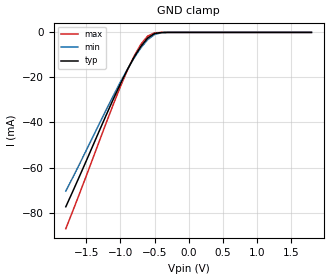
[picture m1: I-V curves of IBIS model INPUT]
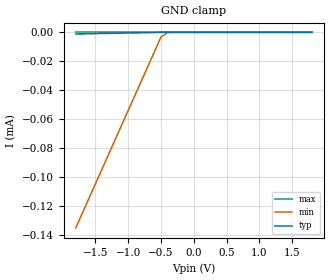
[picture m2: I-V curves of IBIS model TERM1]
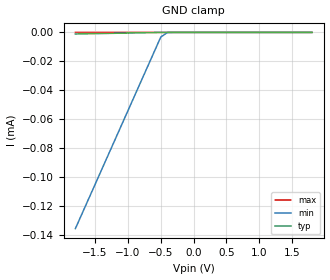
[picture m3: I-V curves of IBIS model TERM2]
|   PERICOM SEMICONDUCTOR CORP
|   IBIS Model of PI2PCIE2412
|   Product Family: 2PCIE
|   TQFN (ZH42) Package
[IBIS Ver] 3.2
[Comment char] |_char
[File Name] pi2pcie2412_zh_18v.ibs
[File Rev] 2.0
[Source] File originated at Pericom Semiconductor Corp.
[Date] 8/9/15
[Disclaimer] (C) Copyright PERICOM Semiconductor Corporation
   All rights reserved
  Pericom Semiconductor Corporation hereby grants the user of
  this IBIS model a non-exclusive, nontransferable license to
  use this IBIS model under the following terms.
  This IBIS model is provided on an "AS IS" basis and Pericom
  makes absolutely no warranty with respect to the information
  contained herein. PERICOM DISCLAIMS AND CUSTOMER WAIVES ALL
  WARRANTIES, EXPRESSED OR IMPLIED, INCLUDING WARRANTIES OF
  MERCHANTABILITY OR FITNESS FOR A PARTICULAR PURPOSE. The
  entire risk as to quality and performance is with the customer.
  Accordingly, in no event shall the company be liable for any
  damages, whether in contract or tort, including any lost
  profits or other incidental, consequential, exemplary, or
  punitive damages arising out of the use or application of the
  IBIS model provided in this package. Further, Pericom reserves
  the right to make changes without notice to any product herein
  to improve reliability, function, or design. Pericom does not
  convey any license under patent rights or any other intellectual
  property rights, including those of third parties.
  The user is granted this license only to use the IBIS model
  and is not granted rights to sell, load, rent, lease or license
  the IBIS model in whole or in part, or in modified form to anyone
  other than user. User may modify the IBIS model to suit its specific
  application but rights to derivative works and such modifications
  shall belong to Pericom.
  Pericom is not obligated to provide maintenance or support
  for the licensed IBIS model.
  Contact Pericom at ATTN: APPLICATION ENGINEERING / IBIS MODELS
  1545 Barber Lane Milpitas, CA 95035 USA.
[Component] PI2PCIE2412
[Manufacturer] Pericom Semiconductor Corp.
[Package]
| variable   typ   min   max
R_pkg   0.06724ohm   0.06412ohm   0.07036ohm
L_pkg   3.83637nH   3.59345nH   3.83637nH
C_pkg   0.37930pF   0.27606pF   0.48254pF
[Pin]  signal_name   model_name   R_pin   L_pin   C_pin
1   GND   GND   0.07036   4.07929nH   0.48254pF
2   A0+   TERM1   0.06958   4.01856nH   0.45673pF
3   A0-   TERM1   0.06880   3.95783nH   0.43092pF
4   GND   GND   0.06802   3.89710nH   0.40511pF
5   VDD   POWER   0.06724   3.83637nH   0.37930pF
6   A1+   TERM1   0.06646   3.77564nH   0.35349pF
7   A1-   TERM1   0.06568   3.71491nH   0.32768pF
8   VDD   POWER   0.06490   3.65418nH   0.30187pF
9   SEL   INPUT   0.06412   3.59345nH   0.27606pF
10   GND   GND   0.06490   3.65418nH   0.30187pF
11   A2+   TERM1   0.06568   3.71491nH   0.32768pF
12   A2-   TERM1   0.06646   3.77564nH   0.35349pF
13   VDD   POWER   0.06724   3.83637nH   0.37930pF
14   GND   GND   0.06802   3.89710nH   0.40511pF
15   A3+   TERM1   0.06880   3.95783nH   0.43092pF
16   A3-   TERM1   0.06958   4.01856nH   0.45673pF
17   GND   GND   0.07036   4.07929nH   0.48254pF
18   VDD   POWER   0.07036   4.07929nH   0.48254pF
19   GND   GND   0.06742   3.84713nH   0.35011pF
20   VDD   POWER   0.06742   3.84713nH   0.35011pF
21   GND   GND   0.07036   4.07929nH   0.48254pF
22   C3-   TERM2   0.07036   4.07929nH   0.48254pF
23   C3+   TERM2   0.06958   4.01856nH   0.45673pF
24   C2-   TERM2   0.06880   3.95783nH   0.43092pF
25   C2+   TERM2   0.06802   3.89710nH   0.40511pF
26   B3-   TERM2   0.06724   3.83637nH   0.37930pF
27   B3+   TERM2   0.06646   3.77564nH   0.35349pF
28   B2-   TERM2   0.06568   3.71491nH   0.32768pF
29   B2+   TERM2   0.06490   3.65418nH   0.30187pF
30   VDD   POWER   0.06412   3.59345nH   0.27606pF
31   C1-   TERM2   0.06490   3.65418nH   0.30187pF
32   C1+   TERM2   0.06568   3.71491nH   0.32768pF
33   C0-   TERM2   0.06646   3.77564nH   0.35349pF
34   C0+   TERM2   0.06724   3.83637nH   0.37930pF
35   B1-   TERM2   0.06802   3.89710nH   0.40511pF
36   B1+   TERM2   0.06880   3.95783nH   0.43092pF
37   B0-   TERM2   0.06958   4.01856nH   0.45673pF
38   B0+   TERM2   0.07036   4.07929nH   0.48254pF
39   GND   GND   0.07036   4.07929nH   0.48254pF
40   VDD   POWER   0.06742   3.84713nH   0.35011pF
41   GND   GND   0.06742   3.84713nH   0.35011pF
42   VDD   POWER   0.07036   4.07929nH   0.48254pF
[Series Switch Groups]
On 1 /
Off 2 /
[Series Pin Mapping]   pin_2   model_name  function_table_group
2   38   SWITCH1   1
3   37   SWITCH1   1
6   36   SWITCH1   1
7   35   SWITCH1   1
11   29   SWITCH1   1
12   28   SWITCH1   1
15   27   SWITCH1   1
16   26   SWITCH1   1
2   34   SWITCH1   2
3   33   SWITCH1   2
6   32   SWITCH1   2
7   31   SWITCH1   2
11   25   SWITCH1   2
12   24   SWITCH1   2
15   23   SWITCH1   2
16   22   SWITCH1   2
|   Model SWITCH1
[Model] SWITCH1
Model_type Series_switch
| variable   typ   min   max
C_comp   2.000pF   1.900pF   2.100pF
[Voltage Range]   1.800V   1.620V   1.980V
[GND Clamp Reference]   0.000V   0.000V   0.000V
[POWER Clamp Reference]   1.800V   1.620V   1.980V
[Temperature Range]   25   -45   85
[On]
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[OFF]
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| Models and submodels in the file (4): INPUT (Input), SWITCH1 (Series_switch), TERM1 (Terminator), TERM2 (Terminator)
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|   Model INPUT
[Model] INPUT
Model_type Input
Vinl = 0.800V
Vinh = 2.000V
| variable   typ   min   max
C_comp   1.200pF   1.100pF   1.300pF
[Voltage Range]   1.800V   1.620V   1.980V
[GND Clamp Reference]   0.000V   0.000V   0.000V
[POWER Clamp Reference]   1.800V   1.620V   1.980V
[Temperature Range]   25   -45   85
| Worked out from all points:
|   GND clamp passes 1 mA (typ) near -0.52 V on its own axis
[GND Clamp]
| Voltage   I(typ)   I(min)   I(max)
-1.8V     -77.42mA   -70.49mA   -87.16mA
-1.6V     -63.94mA   -58.5mA    -71.67mA
-1.2V     -36.16mA   -33.87mA   -39.55mA
-1V       -22.84mA   -22.05mA   -24.09mA
-900mV    -16.68mA   -16.52mA   -16.97mA
-800mV    -11.05mA   -11.41mA   -10.58mA
-700mV    -6.187mA   -6.868mA   -5.263mA
-600mV    -2.494mA   -3.217mA   -1.617mA
-500mV    -532.7uA   -953.5uA   -191.2uA
-400mV    -51.38uA   -151.8uA   -8.195uA
-300mV    -2.895uA   -15.2uA    -172nA
1.8V      494.8pA    12.63nA    29.1pA
[POWER Clamp]
| Voltage   I(typ)   I(min)   I(max)
-1.8V     0A         0A         0A
0V        0A         0A         0A
|   Model TERM1
[Model] TERM1
Model_type Terminator
| variable   typ   min   max
C_comp   1.000pF   0.950pF   1.050pF
[Voltage Range]   1.800V   1.620V   1.980V
[GND Clamp Reference]   0.000V   0.000V   0.000V
[POWER Clamp Reference]   1.800V   1.620V   1.980V
[Temperature Range]   25   -45   85
[GND Clamp]
| Voltage   I(typ)   I(min)   I(max)
-1.8V     -1.106uA   -135.4uA   -523.9pA
-500mV    -22nA      -3.216uA   -29.1pA
-400mV    -509.3pA   -136.8nA   -21.83pA
1.8V      0A         0A         0A
[POWER Clamp]
| Voltage   I(typ)   I(min)   I(max)
-1.8V     0A         0A         0A
0V        0A         0A         0A
|   Model TERM2
[Model] TERM2
Model_type Terminator
| variable   typ   min   max
C_comp   1.000pF   0.950pF   1.050pF
[Voltage Range]   1.800V   1.620V   1.980V
[GND Clamp Reference]   0.000V   0.000V   0.000V
[POWER Clamp Reference]   1.800V   1.620V   1.980V
[Temperature Range]   25   -45   85
[GND Clamp]
| Voltage   I(typ)   I(min)   I(max)
-1.8V     -1.106uA   -135.4uA   -553pA
-500mV    -22nA      -3.204uA   -36.38pA
-400mV    -523.9pA   -136.7nA   -14.55pA
1.8V      0A         0A         0A
[POWER Clamp]
| Voltage   I(typ)   I(min)   I(max)
-1.8V     0A         0A         0A
0V        0A         0A         0A
